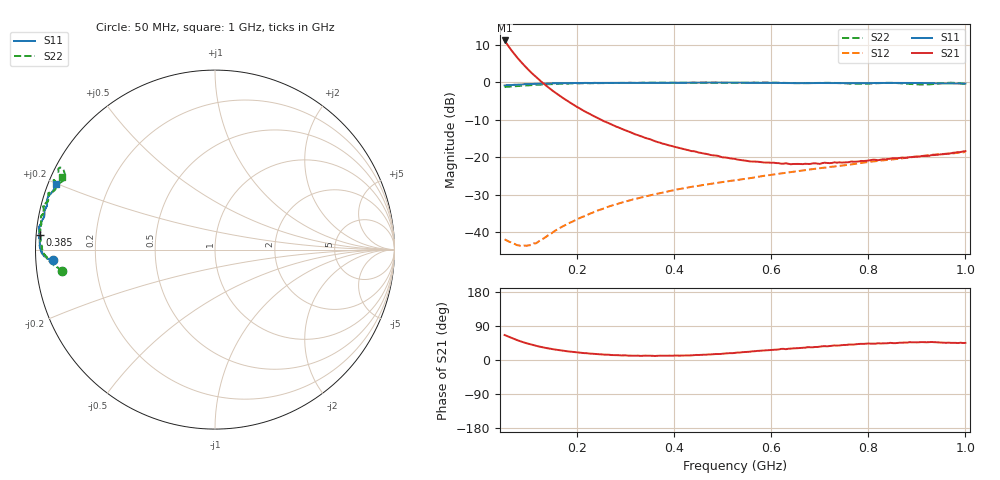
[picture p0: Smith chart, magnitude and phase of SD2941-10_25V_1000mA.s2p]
!Agilent Technologies,E8358A,US42080673,A.04.86
!Agilent E8358A: A.04.86
!Date: Friday, June 09, 2006 14:44:39
!Correction: S11(Full 2 Port SOLT,1,2) S21(Full 2 Port SOLT,1,2) S12(Full 2 Port SOLT,1,2) S22(Full 2 Port SOLT,1,2)
!S2P File: Measurements: S11, S21, S12, S22:
# Hz S  MA  R 50
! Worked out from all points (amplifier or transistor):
!   191 points, 50 MHz to 1 GHz, reference 50 ohm
!   highest |S21| = 11.1 dB at 50 MHz (marker M1)
!   |S21| within 3 dB of that: start of sweep to 66.35 MHz
!   unconditionally stable (mu >= 1): 745.8 MHz to 821 MHz; 870.4 MHz to 958.9 MHz; 985.4 MHz to end of sweep
!   at 205 MHz: K = 0.39, MSG = 14.6 dB, |S12| = -36.1 dB
!   at 525 MHz: K = 0.54, MSG = 2.8 dB, |S12| = -26.1 dB
!   at 1 GHz: K = 1.11, MAG = -1.9 dB, |S12| = -18.6 dB
!   S11 on the Smith chart (normalised r, x): 50 MHz: 0.05, -0.03; 385 MHz: 0.01, +0.04; 1 GHz: 0.02, +0.20
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5e7  0.9037 -176.4  3.584 65.9  0.008087 7.0  0.86 -172.0
5.5e7  0.9111 -176.2  3.199 63.2  0.007775 8.6  0.8675 -172.5
6e7  0.9129 -176.4  2.881 60.3  0.007495 9.8  0.8702 -172.8
6.5e7  0.9146 -176.4  2.602 57.6  0.007335 12.4  0.8773 -173.1
7.5e7  0.9235 -176.6  2.16 52.8  0.006789 19.8  0.8856 -173.6
8e7  0.929 -176.7  1.979 50.4  0.006713 23.2  0.8901 -174.0
9e7  0.9363 -176.8  1.678 46.3  0.006694 31.1  0.9028 -174.4
1.05e8  0.9439 -177.5  1.337 40.7  0.006794 43.3  0.9118 -175.2
1.25e8  0.9546 -178.0  1.023 34.4  0.008011 57.6  0.9282 -176.3
1.5e8  0.9645 -178.8  0.7595 28.2  0.0101 69.7  0.941 -177.7
1.75e8  0.9696 -179.6  0.5872 23.6  0.0125 74.0  0.9542 -179.0
2.1e8  0.9733 179.5  0.4267 18.7  0.01608 77.0  0.9658 179.5
2.8e8  0.976 177.5  0.2559 12.9  0.02351 78.6  0.9733 176.3
3.7e8  0.98 175.7  0.1567 11.4  0.03312 77.7  0.9804 172.9
3.85e8  0.9788 175.2  0.1467 11.2  0.03491 77.3  0.9782 172.2
5.25e8  0.9842 172.2  0.09506 18.9  0.0494 73.6  0.9749 167.6
6.2e8  0.9755 169.9  0.08214 29.2  0.06098 70.8  0.9764 164.9
6.85e8  0.9717 168.3  0.08285 33.5  0.0697 69.4  0.9755 162.1
8.45e8  0.9746 163.7  0.09573 45.3  0.09286 64.8  0.9789 156.9
9.2e8  0.9691 161.6  0.1041 46.8  0.1059 62.5  0.9303 154.0
9.6e8  0.9592 159.7  0.111 45.3  0.1114 60.5  0.9778 152.1
1e9  0.9567 157.5  0.1207 45.2  0.1175 57.0  0.9443 154.7
